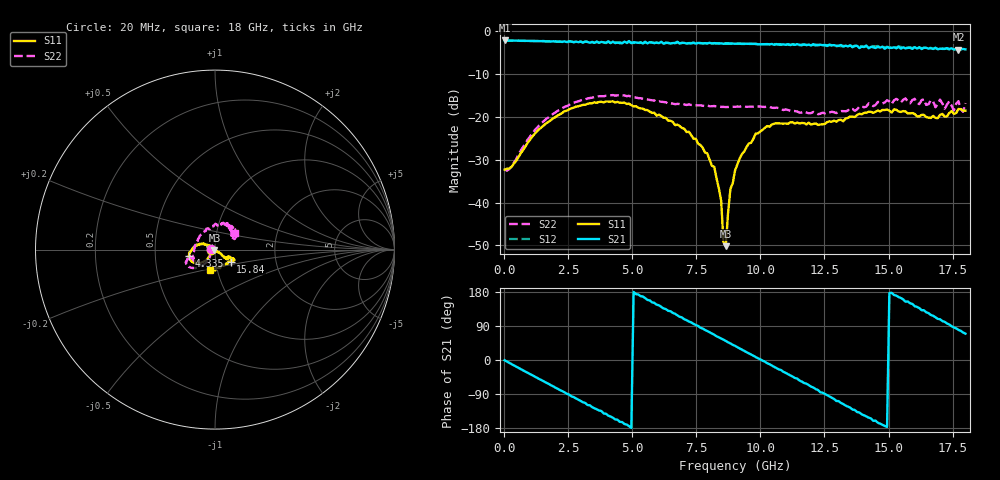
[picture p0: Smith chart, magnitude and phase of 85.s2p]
!Agilent Technologies,N5230A,US43500223,A.07.50.48
!Agilent N5230A: A.07.50.48
!Date: Tuesday, January 12, 2016 19:53:30
!Correction: S11(Full 2 Port(1,2))
!S21(Full 2 Port(1,2))
!S12(Full 2 Port(1,2))
!S22(Full 2 Port(1,2))
!S2P File: Measurements: S11, S21, S12, S22:
# Hz S  dB  R 50
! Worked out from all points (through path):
!   201 points, 20 MHz to 18 GHz, reference 50 ohm
!   highest |S21| = -2.15 dB at 20 MHz (marker M1); lowest = -4.3 dB at 17.73 GHz (marker M2)
!   group delay of S21, straight-line fit = 100 ps
!   lowest |S11| = -50.2 dB at 8.65 GHz (marker M3), VSWR 1.01, Z = 49.7 - j0.13 ohm
!   |S11| at or under -10 dB: start of sweep to end of sweep
!   |S22| runs from -32.6 to -14.9 dB; largest |S21 - S12| = 0.034
!   S11 on the Smith chart (normalised r, x): 20 MHz: 0.95, -0.00; 4.335 GHz: 0.75, -0.06; 15.84 GHz: 1.18, -0.16; 18 GHz: 0.92, -0.21
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2e7  -32.31 -178.4  -2.15 -0.7  -2.15 -0.8  -32.28 178.5
1.5483e9  -21.97 -129.9  -2.28 -56.5  -2.29 -56.7  -20.94 -125.1
3.0766e9  -17.21 -147.3  -2.65 -111.5  -2.59 -111.4  -16.03 -139.8
4.3352e9  -16.63 -165.7  -2.77 -156.7  -2.60 -156.3  -15.04 -152.3
4.8746e9  -16.92 -174.5  -2.29 -174.3  -2.49 -174.2  -15.08 -156.9
6.0433e9  -19.48 165.1  -2.76 144.3  -2.84 143.9  -16.35 -162.9
7.0322e9  -22.79 155.0  -2.72 107.3  -2.79 108.0  -17.09 -162.2
8.2009e9  -31.68 147.9  -2.76 66.6  -2.83 66.3  -17.45 -157.4
8.4706e9  -39.61 161.0  -2.82 56.6  -2.86 56.8  -17.66 -155.3
8.5605e9  -49.27 -163.5  -2.94 53.8  -2.86 53.4  -17.67 -154.0
8.6504e9  -50.20 -154.9  -2.84 50.3  -2.88 50.0  -17.70 -154.5
8.8302e9  -36.82 -34.5  -2.85 43.8  -2.89 43.9  -17.59 -152.3
9.01e9  -32.56 -40.6  -2.92 37.4  -2.89 37.2  -17.65 -151.9
1.02686e10  -22.14 -39.2  -3.00 -8.6  -3.04 -7.8  -17.60 -154.8
1.20666e10  -21.63 -31.0  -3.02 -72.6  -3.17 -73.5  -18.83 158.6
1.3505e10  -19.91 -28.7  -3.30 -125.7  -3.34 -125.6  -17.97 112.1
1.50333e10  -18.57 -27.8  -3.88 176.9  -3.79 177.9  -16.37 68.2
1.58424e10  -19.17 -37.7  -3.86 149.7  -3.71 147.2  -16.82 58.3
1.68313e10  -20.25 -66.8  -3.84 112.9  -3.93 112.7  -17.73 43.1
1.77303e10  -18.15 -96.9  -4.28 79.3  -4.23 78.4  -16.32 33.9
1.79101e10  -18.54 -101.8  -4.12 72.5  -4.19 71.8  -18.81 40.0
1.8e10  -18.53 -104.8  -4.22 69.7  -4.29 68.9  -16.77 40.5
